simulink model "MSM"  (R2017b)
settings: Solver=FixedStepDiscrete  StartTime=0.0  StopTime=10.0  FixedStep=0.01  RelTol=1e-3  EnableMultiTasking=on
undefined symbols (not defined in the file): ASWTYPE_FALSE, ASWTYPE_TRUE, CcMSM_NetWorkRlsTi_ms, CcMSM_PreShutTi_ms, CcMSM_RadySleepFltTi_ms, CcMSM_SelfCheckFltThrhd_numb, CcMSM_ShutdownToSleepTi_ms, CcMSM_ShutdownToStbTi_ms, CcMSM_StandbyRunTime_ms, CcMSM_StbToPreShutDlyTi_ms, Enum_CTCCtrCtlState, Enum_ISPBsicSysMod, Enum_ISPNetWkUpSt, Enum_MSMBMUState, Enum_VDPDriveRqst, MSM_RUNTIME_MS, WAKEUP_DEFAULT
libraries: AIWAYS_Powertrain_BMS_lib x18

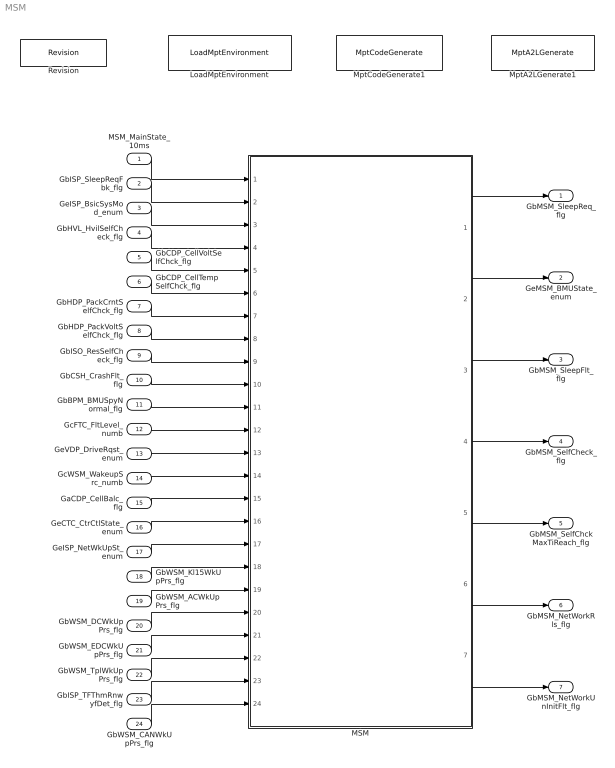
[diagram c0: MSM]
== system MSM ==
  MSM_MainState_10ms : Inport
  GbISP_SleepReqFbk_flg : Inport  Port=2
  GeISP_BsicSysMod_enum : Inport  Port=3
  GbHVL_HvilSelfCheck_flg : Inport  Port=4
  GbCDP_CellVoltSelfChck_flg : Inport  Port=5
  GbCDP_CellTempSelfChck_flg : Inport  Port=6
  GbHDP_PackCrntSelfChck_flg : Inport  Port=7
  GbHDP_PackVoltSelfChck_flg : Inport  Port=8
  GbISO_ResSelfCheck_flg : Inport  Port=9
  GbCSH_CrashFlt_flg : Inport  Port=10
  GbBPM_BMUSpyNormal_flg : Inport  Port=11
  GcFTC_FltLevel_numb : Inport  Port=12
  GeVDP_DriveRqst_enum : Inport  Port=13
  GcWSM_WakeupSrc_numb : Inport  Port=14
  GaCDP_CellBalc_flg : Inport  Port=15
  GeCTC_CtrCtlState_enum : Inport  Port=16
  GeISP_NetWkUpSt_enum : Inport  Port=17
  GbWSM_Kl15WkUpPrs_flg : Inport  Port=18
  GbWSM_ACWkUpPrs_flg : Inport  Port=19
  GbWSM_DCWkUpPrs_flg : Inport  Port=20
  GbWSM_EDCWkUpPrs_flg : Inport  Port=21
  GbWSM_TplWkUpPrs_flg : Inport  Port=22
  GbISP_TFThmRnwyfDet_flg : Inport  Port=23
  GbWSM_CANWkUpPrs_flg : Inport  Port=24
  LoadMptEnvironment : AIWAYS_Powertrain_BMS_lib/Config/LoadMptEnvironment  ProjectName=Comm  SuppierID=NewPlatformUAES
  MSM : Subsystem
  MptA2LGenerate1 : AIWAYS_Powertrain_BMS_lib/Config/MptA2LGenerate  SystemSampleTime=-1
  MptCodeGenerate1 : AIWAYS_Powertrain_BMS_lib/Config/MptCodeGenerate  SystemSampleTime=-1
  Revision : AIWAYS_Powertrain_BMS_lib/Config/Revision  curVersion='M108C103'  newVersion='M108C103'
  GbMSM_SleepReq_flg : Outport
  GeMSM_BMUState_enum : Outport  Port=2
  GbMSM_SleepFlt_flg : Outport  Port=3
  GbMSM_SelfCheck_flg : Outport  Port=4
  GbMSM_SelfChckMaxTiReach_flg : Outport  Port=5
  GbMSM_NetWorkRls_flg : Outport  Port=6
  GbMSM_NetWorkUnInitFlt_flg : Outport  Port=7
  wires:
  MSM_MainState_10ms/1 -> MSM/1(MSM_MainState_10ms)
  GbISP_SleepReqFbk_flg/1 -> MSM/2(GbISP_SleepReqFbk_flg)
  GeISP_BsicSysMod_enum/1 -> MSM/3(GeISP_BsicSysMod_enum)
  GbHVL_HvilSelfCheck_flg/1 -> MSM/4(GbHVL_HvilSelfCheck_flg)
  GbCDP_CellVoltSelfChck_flg/1 -> MSM/5(GbCDP_CellVoltSelfChck_flg)
  GbCDP_CellTempSelfChck_flg/1 -> MSM/6(GbCDP_CellTempSelfChck_flg)
  GbHDP_PackCrntSelfChck_flg/1 -> MSM/7(GbHDP_PackCrntSelfChck_flg)
  GbHDP_PackVoltSelfChck_flg/1 -> MSM/8(GbHDP_PackVoltSelfChck_flg)
  GbISO_ResSelfCheck_flg/1 -> MSM/9(GbISO_ResSelfCheck_flg)
  GbCSH_CrashFlt_flg/1 -> MSM/10(GbCSH_CrashFlt_flg)
  GbBPM_BMUSpyNormal_flg/1 -> MSM/11(GbBPM_BMUSpyNormal_flg)
  GcFTC_FltLevel_numb/1 -> MSM/12(GcFTC_FltLevel_numb)
  GeVDP_DriveRqst_enum/1 -> MSM/13(GeVDP_DriveRqst_enum)
  GcWSM_WakeupSrc_numb/1 -> MSM/14(GcWSM_WakeupSrc_numb)
  GaCDP_CellBalc_flg/1 -> MSM/15(GaCDP_CellBalc_flg)
  GeCTC_CtrCtlState_enum/1 -> MSM/16(GeCTC_CtrCtlState_enum)
  GbWSM_Kl15WkUpPrs_flg/1 -> MSM/18(GbWSM_Kl15WkUpPrs_flg)
  GbWSM_ACWkUpPrs_flg/1 -> MSM/19(GbWSM_ACWkUpPrs_flg)
  GbWSM_DCWkUpPrs_flg/1 -> MSM/20(GbWSM_DCWkUpPrs_flg)
  GbWSM_EDCWkUpPrs_flg/1 -> MSM/21(GbWSM_EDCWkUpPrs_flg)
  MSM/1(GbMSM_SleepReq_flg) -> GbMSM_SleepReq_flg/1
  MSM/2(GeMSM_BMUState_enum) -> GeMSM_BMUState_enum/1
  MSM/3(GbMSM_SleepFlt_flg) -> GbMSM_SleepFlt_flg/1
  MSM/4(GbMSM_SelfCheck_flg) -> GbMSM_SelfCheck_flg/1
  MSM/5(GbMSM_SelfChckMaxTiReach_flg) -> GbMSM_SelfChckMaxTiReach_flg/1
  MSM/6(GbMSM_NetWorkRls_flg) -> GbMSM_NetWorkRls_flg/1
  MSM/7(GbMSM_NetWorkUnInitFlt_flg) -> GbMSM_NetWorkUnInitFlt_flg/1
  GbWSM_TplWkUpPrs_flg/1 -> MSM/22(GbWSM_TplWkUpPrs_flg)
  GbISP_TFThmRnwyfDet_flg/1 -> MSM/23(GbISP_TFThmRnwyfDet_flg)
  GbWSM_CANWkUpPrs_flg/1 -> MSM/24(GbWSM_CANWkUpPrs_flg)
  GeISP_NetWkUpSt_enum/1 -> MSM/17(GeISP_NetWkUpSt_enum)

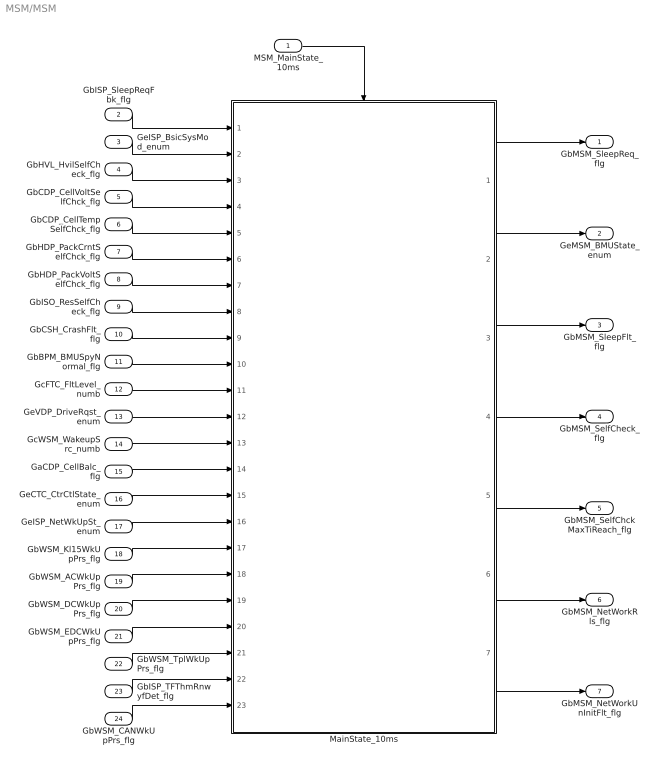
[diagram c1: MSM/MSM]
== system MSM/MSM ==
  MSM_MainState_10ms : Inport
  GbISP_SleepReqFbk_flg : Inport  Port=2
  GeISP_BsicSysMod_enum : Inport  Port=3
  GbHVL_HvilSelfCheck_flg : Inport  Port=4
  GbCDP_CellVoltSelfChck_flg : Inport  Port=5
  GbCDP_CellTempSelfChck_flg : Inport  Port=6
  GbHDP_PackCrntSelfChck_flg : Inport  Port=7
  GbHDP_PackVoltSelfChck_flg : Inport  Port=8
  GbISO_ResSelfCheck_flg : Inport  Port=9
  GbCSH_CrashFlt_flg : Inport  Port=10
  GbBPM_BMUSpyNormal_flg : Inport  Port=11
  GcFTC_FltLevel_numb : Inport  Port=12
  GeVDP_DriveRqst_enum : Inport  Port=13
  GcWSM_WakeupSrc_numb : Inport  Port=14
  GaCDP_CellBalc_flg : Inport  Port=15
  GeCTC_CtrCtlState_enum : Inport  Port=16
  GeISP_NetWkUpSt_enum : Inport  Port=17
  GbWSM_Kl15WkUpPrs_flg : Inport  Port=18
  GbWSM_ACWkUpPrs_flg : Inport  Port=19
  GbWSM_DCWkUpPrs_flg : Inport  Port=20
  GbWSM_EDCWkUpPrs_flg : Inport  Port=21
  GbWSM_TplWkUpPrs_flg : Inport  Port=22
  GbISP_TFThmRnwyfDet_flg : Inport  Port=23
  GbWSM_CANWkUpPrs_flg : Inport  Port=24
  MainState_10ms : Subsystem
  GbMSM_SleepReq_flg : Outport
  GeMSM_BMUState_enum : Outport  Port=2
  GbMSM_SleepFlt_flg : Outport  Port=3
  GbMSM_SelfCheck_flg : Outport  Port=4
  GbMSM_SelfChckMaxTiReach_flg : Outport  Port=5
  GbMSM_NetWorkRls_flg : Outport  Port=6
  GbMSM_NetWorkUnInitFlt_flg : Outport  Port=7
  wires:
  MSM_MainState_10ms/1 -> MainState_10ms/Trigger
  GbISP_SleepReqFbk_flg/1 -> MainState_10ms/1(GbISP_SleepReqFbk_flg)
  GeISP_BsicSysMod_enum/1 -> MainState_10ms/2(GeISP_BsicSysMod_enum)
  GbHVL_HvilSelfCheck_flg/1 -> MainState_10ms/3(GbHVL_HvilSelfCheck_flg)
  GbCDP_CellVoltSelfChck_flg/1 -> MainState_10ms/4(GbCDP_CellVoltSelfChck_flg)
  GbCDP_CellTempSelfChck_flg/1 -> MainState_10ms/5(GbCDP_CellTempSelfChck_flg)
  GbHDP_PackCrntSelfChck_flg/1 -> MainState_10ms/6(GbHDP_PackCrntSelfChck_flg)
  GbHDP_PackVoltSelfChck_flg/1 -> MainState_10ms/7(GbHDP_PackVoltSelfChck_flg)
  GbISO_ResSelfCheck_flg/1 -> MainState_10ms/8(GbISO_ResSelfCheck_flg)
  GbCSH_CrashFlt_flg/1 -> MainState_10ms/9(GbCSH_CrashFlt_flg)
  GbBPM_BMUSpyNormal_flg/1 -> MainState_10ms/10(GbBPM_BMUSpyNormal_flg)
  GcFTC_FltLevel_numb/1 -> MainState_10ms/11(GcFTC_FltLevel_numb)
  GeVDP_DriveRqst_enum/1 -> MainState_10ms/12(GeVDP_DriveRqst_enum)
  GcWSM_WakeupSrc_numb/1 -> MainState_10ms/13(GcWSM_WakeupSrc_numb)
  GaCDP_CellBalc_flg/1 -> MainState_10ms/14(GaCDP_CellBalc_flg)
  GeCTC_CtrCtlState_enum/1 -> MainState_10ms/15(GeCTC_CtrCtlState_enum)
  GbWSM_Kl15WkUpPrs_flg/1 -> MainState_10ms/17(GbWSM_Kl15WkUpPrs_flg)
  GbWSM_ACWkUpPrs_flg/1 -> MainState_10ms/18(GbWSM_ACWkUpPrs_flg)
  GbWSM_DCWkUpPrs_flg/1 -> MainState_10ms/19(GbWSM_DCWkUpPrs_flg)
  GbWSM_EDCWkUpPrs_flg/1 -> MainState_10ms/20(GbWSM_EDCWkUpPrs_flg)
  MainState_10ms/4(GbMSM_SelfCheck_flg) -> GbMSM_SelfCheck_flg/1
  MainState_10ms/7(GbMSM_NetWorkUnInitFlt_flg) -> GbMSM_NetWorkUnInitFlt_flg/1
  MainState_10ms/6(GbMSM_NetWorkRls_flg) -> GbMSM_NetWorkRls_flg/1
  MainState_10ms/2(GeMSM_BMUState_enum) -> GeMSM_BMUState_enum/1
  MainState_10ms/3(GbMSM_SleepFlt_flg) -> GbMSM_SleepFlt_flg/1
  MainState_10ms/1(GbMSM_SleepReq_flg) -> GbMSM_SleepReq_flg/1
  MainState_10ms/5(GbMSM_SelfChckMaxTiReach_flg) -> GbMSM_SelfChckMaxTiReach_flg/1
  GbWSM_TplWkUpPrs_flg/1 -> MainState_10ms/21(GbWSM_TplWkUpPrs_flg)
  GbISP_TFThmRnwyfDet_flg/1 -> MainState_10ms/22(GbISP_TFThmRnwyfDet_flg)
  GbWSM_CANWkUpPrs_flg/1 -> MainState_10ms/23(GbWSM_CANWkUpPrs_flg)
  GeISP_NetWkUpSt_enum/1 -> MainState_10ms/16(GeISP_NetWkUpSt_enum)

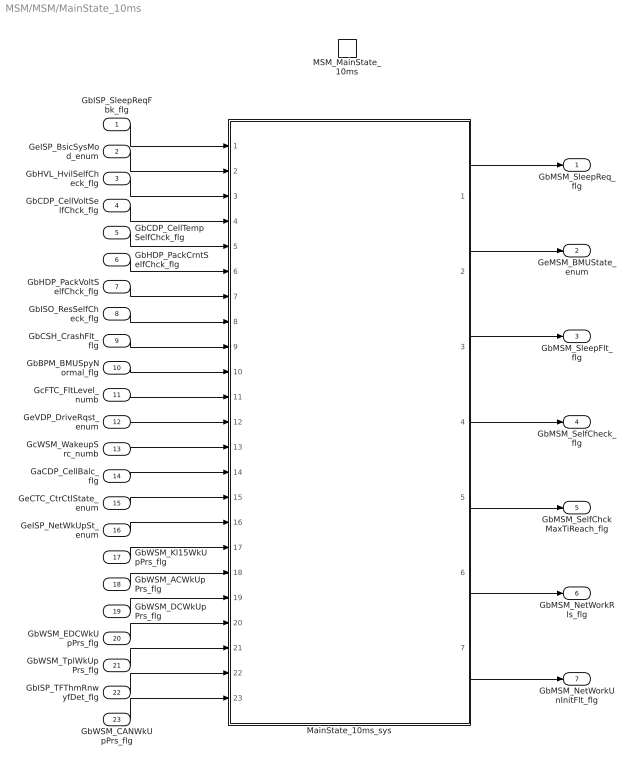
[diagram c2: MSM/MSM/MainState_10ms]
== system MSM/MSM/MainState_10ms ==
  GbISP_SleepReqFbk_flg : Inport
  GeISP_BsicSysMod_enum : Inport  Port=2
  GbHVL_HvilSelfCheck_flg : Inport  Port=3
  GbCDP_CellVoltSelfChck_flg : Inport  Port=4
  GbCDP_CellTempSelfChck_flg : Inport  Port=5
  GbHDP_PackCrntSelfChck_flg : Inport  Port=6
  GbHDP_PackVoltSelfChck_flg : Inport  Port=7
  GbISO_ResSelfCheck_flg : Inport  Port=8
  GbCSH_CrashFlt_flg : Inport  Port=9
  GbBPM_BMUSpyNormal_flg : Inport  Port=10
  GcFTC_FltLevel_numb : Inport  Port=11
  GeVDP_DriveRqst_enum : Inport  Port=12
  GcWSM_WakeupSrc_numb : Inport  Port=13
  GaCDP_CellBalc_flg : Inport  Port=14
  GeCTC_CtrCtlState_enum : Inport  Port=15
  GeISP_NetWkUpSt_enum : Inport  Port=16
  GbWSM_Kl15WkUpPrs_flg : Inport  Port=17
  GbWSM_ACWkUpPrs_flg : Inport  Port=18
  GbWSM_DCWkUpPrs_flg : Inport  Port=19
  GbWSM_EDCWkUpPrs_flg : Inport  Port=20
  GbWSM_TplWkUpPrs_flg : Inport  Port=21
  GbISP_TFThmRnwyfDet_flg : Inport  Port=22
  GbWSM_CANWkUpPrs_flg : Inport  Port=23
  MSM_MainState_10ms : TriggerPort  TriggerType=function-call  VariantControl=(inherit)
  MainState_10ms_sys : Subsystem
  GbMSM_SleepReq_flg : Outport
  GeMSM_BMUState_enum : Outport  Port=2
  GbMSM_SleepFlt_flg : Outport  Port=3
  GbMSM_SelfCheck_flg : Outport  Port=4
  GbMSM_SelfChckMaxTiReach_flg : Outport  Port=5
  GbMSM_NetWorkRls_flg : Outport  Port=6
  GbMSM_NetWorkUnInitFlt_flg : Outport  Port=7
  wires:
  GbISP_SleepReqFbk_flg/1 -> MainState_10ms_sys/1(GbISP_SleepReqFbk_flg)
  GeISP_BsicSysMod_enum/1 -> MainState_10ms_sys/2(GeISP_BsicSysMod_enum)
  GbHVL_HvilSelfCheck_flg/1 -> MainState_10ms_sys/3(GbHVL_HvilSelfCheck_flg)
  GbCDP_CellVoltSelfChck_flg/1 -> MainState_10ms_sys/4(GbCDP_CellVoltSelfChck_flg)
  GbCDP_CellTempSelfChck_flg/1 -> MainState_10ms_sys/5(GbCDP_CellTempSelfChck_flg)
  GbHDP_PackCrntSelfChck_flg/1 -> MainState_10ms_sys/6(GbHDP_PackCrntSelfChck_flg)
  GbHDP_PackVoltSelfChck_flg/1 -> MainState_10ms_sys/7(GbHDP_PackVoltSelfChck_flg)
  GbISO_ResSelfCheck_flg/1 -> MainState_10ms_sys/8(GbISO_ResSelfCheck_flg)
  GbCSH_CrashFlt_flg/1 -> MainState_10ms_sys/9(GbCSH_CrashFlt_flg)
  GbBPM_BMUSpyNormal_flg/1 -> MainState_10ms_sys/10(GbBPM_BMUSpyNormal_flg)
  GcFTC_FltLevel_numb/1 -> MainState_10ms_sys/11(GcFTC_FltLevel_numb)
  GeVDP_DriveRqst_enum/1 -> MainState_10ms_sys/12(GeVDP_DriveRqst_enum)
  GcWSM_WakeupSrc_numb/1 -> MainState_10ms_sys/13(GcWSM_WakeupSrc_numb)
  GaCDP_CellBalc_flg/1 -> MainState_10ms_sys/14(GaCDP_CellBalc_flg)
  GeCTC_CtrCtlState_enum/1 -> MainState_10ms_sys/15(GeCTC_CtrCtlState_enum)
  GbWSM_Kl15WkUpPrs_flg/1 -> MainState_10ms_sys/17(GbWSM_Kl15WkUpPrs_flg)
  GbWSM_ACWkUpPrs_flg/1 -> MainState_10ms_sys/18(GbWSM_ACWkUpPrs_flg)
  GbWSM_DCWkUpPrs_flg/1 -> MainState_10ms_sys/19(GbWSM_DCWkUpPrs_flg)
  GbWSM_EDCWkUpPrs_flg/1 -> MainState_10ms_sys/20(GbWSM_EDCWkUpPrs_flg)
  MainState_10ms_sys/1(GbMSM_SleepReq_flg) -> GbMSM_SleepReq_flg/1
  MainState_10ms_sys/2(GeMSM_BMUState_enum) -> GeMSM_BMUState_enum/1
  MainState_10ms_sys/3(GbMSM_SleepFlt_flg) -> GbMSM_SleepFlt_flg/1
  MainState_10ms_sys/4(GbMSM_SelfCheck_flg) -> GbMSM_SelfCheck_flg/1
  MainState_10ms_sys/5(GbMSM_SelfChckMaxTiReach_flg) -> GbMSM_SelfChckMaxTiReach_flg/1
  MainState_10ms_sys/6(GbMSM_NetWorkRls_flg) -> GbMSM_NetWorkRls_flg/1
  MainState_10ms_sys/7(GbMSM_NetWorkUnInitFlt_flg) -> GbMSM_NetWorkUnInitFlt_flg/1
  GbWSM_TplWkUpPrs_flg/1 -> MainState_10ms_sys/21(GbWSM_TplWkUpPrs_flg)
  GbISP_TFThmRnwyfDet_flg/1 -> MainState_10ms_sys/22(GbISP_TFThmRnwyfDet_flg)
  GbWSM_CANWkUpPrs_flg/1 -> MainState_10ms_sys/23(GbWSM_CANWkUpPrs_flg)
  GeISP_NetWkUpSt_enum/1 -> MainState_10ms_sys/16(GeISP_NetWkUpSt_enum)

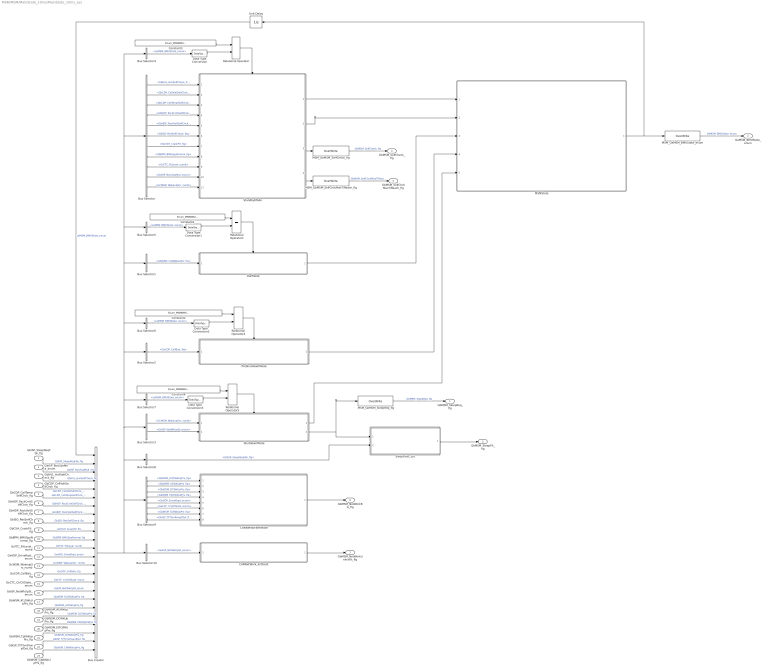
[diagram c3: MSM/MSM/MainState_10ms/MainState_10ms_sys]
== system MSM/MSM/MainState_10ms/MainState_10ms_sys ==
  GbISP_SleepReqFbk_flg : Inport
  GeISP_BsicSysMod_enum : Inport  Port=2
  GbHVL_HvilSelfCheck_flg : Inport  Port=3
  GbCDP_CellVoltSelfChck_flg : Inport  Port=4
  GbCDP_CellTempSelfChck_flg : Inport  Port=5
  GbHDP_PackCrntSelfChck_flg : Inport  Port=6
  GbHDP_PackVoltSelfChck_flg : Inport  Port=7
  GbISO_ResSelfCheck_flg : Inport  Port=8
  GbCSH_CrashFlt_flg : Inport  Port=9
  GbBPM_BMUSpyNormal_flg : Inport  Port=10
  GcFTC_FltLevel_numb : Inport  Port=11
  GeVDP_DriveRqst_enum : Inport  Port=12
  GcWSM_WakeupSrc_numb : Inport  Port=13
  GaCDP_CellBalc_flg : Inport  Port=14
  GeCTC_CtrCtlState_enum : Inport  Port=15
  GeISP_NetWkUpSt_enum : Inport  Port=16
  GbWSM_Kl15WkUpPrs_flg : Inport  Port=17
  GbWSM_ACWkUpPrs_flg : Inport  Port=18
  GbWSM_DCWkUpPrs_flg : Inport  Port=19
  GbWSM_EDCWkUpPrs_flg : Inport  Port=20
  GbWSM_TplWkUpPrs_flg : Inport  Port=21
  GbISP_TFThmRnwyfDet_flg : Inport  Port=22
  GbWSM_CANWkUpPrs_flg : Inport  Port=23
  Bus Creator : BusCreator  Inputs=24
  Bus Selector : BusSelector  OutputSignals=GbHVL_HvilSelfCheck_flg,GbCDP_CellVoltSelfChck_flg,GbCDP_CellTempSelfChck_flg,GbHDP_PackCrntSelfChck_flg,GbHDP_PackVoltSelfChck_flg,GbISO_ResSelfCheck_flg,GbCSH_CrashFlt_flg,GbBPM_BMUSpyNormal_flg,GcFTC_FltLevel_numb,GeISP_BsicSysMod_enum,GcWSM_WakeupSrc_numb
  Bus Selector1 : BusSelector  OutputSignals=GbWSM_CANWkUpPrs_flg
  Bus Selector10 : BusSelector  OutputSignals=GeISP_NetWkUpSt_enum
  Bus Selector2 : BusSelector  OutputSignals=GaCDP_CellBalc_flg
  Bus Selector3 : BusSelector  OutputSignals=GcWSM_WakeupSrc_numb,GeISP_NetWkUpSt_enum
  Bus Selector{4..7} (4 alike) : BusSelector  OutputSignals=LeMSM_BMUState_enum
  Bus Selector8 : BusSelector  OutputSignals=GbISP_SleepReqFbk_flg
  Bus Selector9 : BusSelector  OutputSignals=GbWSM_Kl15WkUpPrs_flg,GbWSM_ACWkUpPrs_flg,GbWSM_DCWkUpPrs_flg,GbWSM_EDCWkUpPrs_flg,GeVDP_DriveRqst_enum,GeCTC_CtrCtlState_enum,GbWSM_TplWkUpPrs_flg,GbISP_TFThmRnwyfDet_flg
  CANNetWorkRelease : Subsystem
  CANNetWork_InitFault : Subsystem
  Constant1 : Constant  Value=Enum_MSMBMUState.Enum_MSMBMUState_Run
  Constant2 : Constant  Value=Enum_MSMBMUState.Enum_MSMBMUState_PreShutdown
  Constant3 : Constant  Value=Enum_MSMBMUState.Enum_MSMBMUState_Standby
  Constant4 : Constant  Value=Enum_MSMBMUState.Enum_MSMBMUState_Shutdown
  Data Type Conversion{,1..3} (4 alike) : DataTypeConversion
  MSMState : Stateflow chart  TreatAsAtomicUnit=on
  MSM_GbMSM_SelfChckMaxTiReach_flg : AIWAYS_Powertrain_BMS_lib/Signals/OverWrite  OverWrite_Value=CbMSM_SelfChckMaxTiReachOvr_flg  OverWrite_flag=CbMSM_SelfChckMaxTiReachOvrSwt_flg
  MSM_GbMSM_SelfCheck_flg : AIWAYS_Powertrain_BMS_lib/Signals/OverWrite  OverWrite_Value=CbMSM_SelfCheckOvr_flg  OverWrite_flag=CbMSM_SelfCheckOvrSwt_flg
  MSM_GbMSM_SleepReq_flg : AIWAYS_Powertrain_BMS_lib/Signals/OverWrite  OverWrite_Value=CbMSM_SleepReqOvr_flg  OverWrite_flag=CbMSM_SleepReqOvrSwt_flg
  MSM_GeMSM_BMUState_enum : AIWAYS_Powertrain_BMS_lib/Signals/OverWrite  OverWrite_Value=CeMSM_BMUStateOvr_enum  OverWrite_flag=CbMSM_BMUStateOvrSwt_flg
  PreShutdownMode : Subsystem  TreatAsAtomicUnit=on
  Relational Operator{,1,4..5} (4 alike) : RelationalOperator  Operator===  OutDataTypeStr=boolean
  RunMode : Subsystem  TreatAsAtomicUnit=on
  ShutdownMode : Subsystem  TreatAsAtomicUnit=on
  SleepFault_sys : Subsystem
  StandbyMode : Subsystem  TreatAsAtomicUnit=on
  Unit Delay : UnitDelay  SampleTime=-1
  GbMSM_SleepReq_flg : Outport
  GeMSM_BMUState_enum : Outport  Port=2
  GbMSM_SleepFlt_flg : Outport  Port=3
  GbMSM_SelfCheck_flg : Outport  Port=4
  GbMSM_SelfChckMaxTiReach_flg : Outport  Port=5
  GbMSM_NetWorkRls_flg : Outport  Port=6
  GbMSM_NetWorkUnInitFlt_flg : Outport  Port=7
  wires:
  GbISP_SleepReqFbk_flg/1 -> Bus Creator/2  "GbISP_SleepReqFbk_flg"
  GeISP_BsicSysMod_enum/1 -> Bus Creator/3  "GeISP_BsicSysMod_enum"
  GbHVL_HvilSelfCheck_flg/1 -> Bus Creator/4  "GbHVL_HvilSelfCheck_flg"
  GbCDP_CellVoltSelfChck_flg/1 -> Bus Creator/5  "GbCDP_CellVoltSelfChck_flg"
  GbCDP_CellTempSelfChck_flg/1 -> Bus Creator/6  "GbCDP_CellTempSelfChck_flg"
  GbHDP_PackCrntSelfChck_flg/1 -> Bus Creator/7  "GbHDP_PackCrntSelfChck_flg"
  GbHDP_PackVoltSelfChck_flg/1 -> Bus Creator/8  "GbHDP_PackVoltSelfChck_flg"
  GbISO_ResSelfCheck_flg/1 -> Bus Creator/9  "GbISO_ResSelfCheck_flg"
  GbCSH_CrashFlt_flg/1 -> Bus Creator/10  "GbCSH_CrashFlt_flg"
  GbBPM_BMUSpyNormal_flg/1 -> Bus Creator/11  "GbBPM_BMUSpyNormal_flg"
  GcFTC_FltLevel_numb/1 -> Bus Creator/12  "GcFTC_FltLevel_numb"
  GeVDP_DriveRqst_enum/1 -> Bus Creator/13  "GeVDP_DriveRqst_enum"
  GcWSM_WakeupSrc_numb/1 -> Bus Creator/14  "GcWSM_WakeupSrc_numb"
  GaCDP_CellBalc_flg/1 -> Bus Creator/15  "GaCDP_CellBalc_flg"
  GeCTC_CtrCtlState_enum/1 -> Bus Creator/16  "GeCTC_CtrCtlState_enum"
  Bus Creator/1 -> Bus Selector8/1, Bus Selector4/1, Bus Selector/1, Bus Selector5/1, Bus Selector1/1, Bus Selector6/1, Bus Selector2/1, Bus Selector7/1, Bus Selector3/1, Bus Selector9/1, Bus Selector10/1
  Bus Selector2/1 -> PreShutdownMode/1(GaCDP_CellBalc_flg)  "<GaCDP_CellBalc_flg>"
  Bus Selector3/1 -> ShutdownMode/1(GcWSM_WakeupSrc_numb)  "<GcWSM_WakeupSrc_numb>"
  StandbyMode/1(LbMSM_StandbyToRun_flg) -> MSMState/1(LbMSM_StandbyToRun_flg)
  StandbyMode/2(LbMSM_StbToPreShut_flg) -> MSMState/2(LbMSM_StbToPreShut_flg)
  RunMode/1(LbMSM_RunToPreShut_flg) -> MSMState/3(LbMSM_RunToPreShut_flg)
  PreShutdownMode/1(LbMSM_PreShutToShut_flg) -> MSMState/4(LbMSM_PreShutToShut_flg)
  ShutdownMode/1(LbMSM_ShutdownToStb_flg) -> MSMState/5(LbMSM_ShutdownToStb_flg)
  MSMState/1(GeMSM_BMUState_enum) -> Unit Delay/1, MSM_GeMSM_BMUState_enum/1
  Relational Operator/1 -> StandbyMode/Enable
  Unit Delay/1 -> Bus Creator/1  "LeMSM_BMUState_enum"
  Constant3/1 -> Relational Operator/1
  Bus Selector4/1 -> Data Type Conversion/1  "<LeMSM_BMUState_enum>"
  Data Type Conversion/1 -> Relational Operator/2
  Bus Selector5/1 -> Data Type Conversion1/1  "<LeMSM_BMUState_enum>"
  Constant1/1 -> Relational Operator1/1
  Relational Operator1/1 -> RunMode/Enable
  Data Type Conversion1/1 -> Relational Operator1/2
  Relational Operator4/1 -> PreShutdownMode/Enable
  Bus Selector6/1 -> Data Type Conversion2/1  "<LeMSM_BMUState_enum>"
  Constant2/1 -> Relational Operator4/1
  Data Type Conversion2/1 -> Relational Operator4/2
  Relational Operator5/1 -> ShutdownMode/Enable
  Bus Selector7/1 -> Data Type Conversion3/1  "<LeMSM_BMUState_enum>"
  Constant4/1 -> Relational Operator5/1
  Data Type Conversion3/1 -> Relational Operator5/2
  MSM_GeMSM_BMUState_enum/1 -> GeMSM_BMUState_enum/1  "GeMSM_BMUState_enum"
  Bus Selector/1 -> StandbyMode/1(GbHVL_HvilSelfCheck_flg)  "<GbHVL_HvilSelfCheck_flg>"
  Bus Selector/2 -> StandbyMode/2(GbCDP_CellVoltSelfChck_flg)  "<GbCDP_CellVoltSelfChck_flg>"
  Bus Selector/3 -> StandbyMode/3(GbCDP_CellTempSelfChck_flg)  "<GbCDP_CellTempSelfChck_flg>"
  Bus Selector/4 -> StandbyMode/4(GbHDP_PackCrntSelfChck_flg)  "<GbHDP_PackCrntSelfChck_flg>"
  Bus Selector/5 -> StandbyMode/5(GbHDP_PackVoltSelfChck_flg)  "<GbHDP_PackVoltSelfChck_flg>"
  Bus Selector/6 -> StandbyMode/6(GbISO_ResSelfCheck_flg)  "<GbISO_ResSelfCheck_flg>"
  Bus Selector/7 -> StandbyMode/7(GbCSH_CrashFlt_flg)  "<GbCSH_CrashFlt_flg>"
  Bus Selector/8 -> StandbyMode/8(GbBPM_BMUSpyNormal_flg)  "<GbBPM_BMUSpyNormal_flg>"
  Bus Selector/9 -> StandbyMode/9(GcFTC_FltLevel_numb)  "<GcFTC_FltLevel_numb>"
  Bus Selector/10 -> StandbyMode/10(GeISP_BsicSysMod_enum)  "<GeISP_BsicSysMod_enum>"
  Bus Selector/11 -> StandbyMode/11(GcWSM_WakeupSrc_numb)  "<GcWSM_WakeupSrc_numb>"
  Bus Selector3/2 -> ShutdownMode/2(GeISP_NetWkUpSt_enum)  "<GeISP_NetWkUpSt_enum>"
  MSM_GbMSM_SleepReq_flg/1 -> GbMSM_SleepReq_flg/1  "GbMSM_SleepReq_flg"
  ShutdownMode/2(LbMSM_SleepReq_flg) -> SleepFault_sys/1(LbMSM_SleepReq_flg), MSM_GbMSM_SleepReq_flg/1
  SleepFault_sys/1(GbMSM_SleepFlt_flg) -> GbMSM_SleepFlt_flg/1
  Bus Selector8/1 -> SleepFault_sys/2(GbISP_SleepReqFbk_flg)  "<GbISP_SleepReqFbk_flg>"
  MSM_GbMSM_SelfCheck_flg/1 -> GbMSM_SelfCheck_flg/1  "GbMSM_SelfCheck_flg"
  StandbyMode/3(LbMSM_SelfCheck_flg) -> MSM_GbMSM_SelfCheck_flg/1
  MSM_GbMSM_SelfChckMaxTiReach_flg/1 -> GbMSM_SelfChckMaxTiReach_flg/1  "GbMSM_SelfChckMaxTiReach_flg"
  StandbyMode/4(LbMSM_SelfChckMaxTiReach_flg) -> MSM_GbMSM_SelfChckMaxTiReach_flg/1
  Bus Selector1/1 -> RunMode/1(GbWSM_CANWkUpPrs_flg)  "<GbWSM_CANWkUpPrs_flg>"
  GbWSM_Kl15WkUpPrs_flg/1 -> Bus Creator/18  "GbWSM_Kl15WkUpPrs_flg"
  GbWSM_ACWkUpPrs_flg/1 -> Bus Creator/19  "GbWSM_ACWkUpPrs_flg"
  GbWSM_DCWkUpPrs_flg/1 -> Bus Creator/20  "GbWSM_DCWkUpPrs_flg"
  GbWSM_EDCWkUpPrs_flg/1 -> Bus Creator/21  "GbWSM_EDCWkUpPrs_flg"
  CANNetWorkRelease/1(GbMSM_NetWorkRls_flg) -> GbMSM_NetWorkRls_flg/1
  Bus Selector10/1 -> CANNetWork_InitFault/1(GeISP_NetWkUpSt_enum)  "<GeISP_NetWkUpSt_enum>"
  CANNetWork_InitFault/1(GbMSM_NetWorkUnInitFlt_flg) -> GbMSM_NetWorkUnInitFlt_flg/1
  Bus Selector9/1 -> CANNetWorkRelease/1(GbWSM_Kl15WkUpPrs_flg)  "<GbWSM_Kl15WkUpPrs_flg>"
  Bus Selector9/2 -> CANNetWorkRelease/2(GbWSM_ACWkUpPrs_flg)  "<GbWSM_ACWkUpPrs_flg>"
  Bus Selector9/3 -> CANNetWorkRelease/3(GbWSM_DCWkUpPrs_flg)  "<GbWSM_DCWkUpPrs_flg>"
  Bus Selector9/4 -> CANNetWorkRelease/4(GbWSM_EDCWkUpPrs_flg)  "<GbWSM_EDCWkUpPrs_flg>"
  Bus Selector9/5 -> CANNetWorkRelease/5(GeVDP_DriveRqst_enum)  "<GeVDP_DriveRqst_enum>"
  Bus Selector9/6 -> CANNetWorkRelease/6(GeCTC_CtrCtlState_enum)  "<GeCTC_CtrCtlState_enum>"
  GbWSM_TplWkUpPrs_flg/1 -> Bus Creator/22  "GbWSM_TplWkUpPrs_flg"
  GbISP_TFThmRnwyfDet_flg/1 -> Bus Creator/23  "GbISP_TFThmRnwyfDet_flg"
  Bus Selector9/7 -> CANNetWorkRelease/7(GbWSM_TplWkUpPrs_flg)  "<GbWSM_TplWkUpPrs_flg>"
  Bus Selector9/8 -> CANNetWorkRelease/8(GbISP_TFThmRnwyfDet_flg)  "<GbISP_TFThmRnwyfDet_flg>"
  GbWSM_CANWkUpPrs_flg/1 -> Bus Creator/24  "GbWSM_CANWkUpPrs_flg"
  GeISP_NetWkUpSt_enum/1 -> Bus Creator/17  "GeISP_NetWkUpSt_enum"

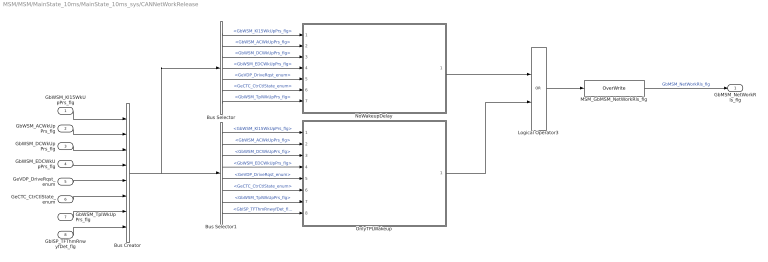
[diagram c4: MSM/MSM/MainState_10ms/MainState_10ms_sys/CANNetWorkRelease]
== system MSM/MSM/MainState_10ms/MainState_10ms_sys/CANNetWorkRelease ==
  GbWSM_Kl15WkUpPrs_flg : Inport
  GbWSM_ACWkUpPrs_flg : Inport  Port=2
  GbWSM_DCWkUpPrs_flg : Inport  Port=3
  GbWSM_EDCWkUpPrs_flg : Inport  Port=4
  GeVDP_DriveRqst_enum : Inport  Port=5
  GeCTC_CtrCtlState_enum : Inport  Port=6
  GbWSM_TplWkUpPrs_flg : Inport  Port=7
  GbISP_TFThmRnwyfDet_flg : Inport  Port=8
  Bus Creator : BusCreator  Inputs=8
  Bus Selector : BusSelector  OutputSignals=GbWSM_Kl15WkUpPrs_flg,GbWSM_ACWkUpPrs_flg,GbWSM_DCWkUpPrs_flg,GbWSM_EDCWkUpPrs_flg,GeVDP_DriveRqst_enum,GeCTC_CtrCtlState_enum,GbWSM_TplWkUpPrs_flg
  Bus Selector1 : BusSelector  OutputSignals=GbWSM_Kl15WkUpPrs_flg,GbWSM_ACWkUpPrs_flg,GbWSM_DCWkUpPrs_flg,GbWSM_EDCWkUpPrs_flg,GeVDP_DriveRqst_enum,GeCTC_CtrCtlState_enum,GbWSM_TplWkUpPrs_flg,GbISP_TFThmRnwyfDet_flg
  Logical Operator3 : Logic  Operator=OR  AllPortsSameDT=off  OutDataTypeStr=boolean
  MSM_GbMSM_NetWorkRls_flg : AIWAYS_Powertrain_BMS_lib/Signals/OverWrite  OverWrite_Value=CbMSM_NetWorkRlsOvr_flg  OverWrite_flag=CbMSM_NetWorkRlsOvrSwt_flg
  NoWakeupDelay : Subsystem
  OnlyTPLWakeup : Subsystem
  GbMSM_NetWorkRls_flg : Outport
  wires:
  Logical Operator3/1 -> MSM_GbMSM_NetWorkRls_flg/1
  MSM_GbMSM_NetWorkRls_flg/1 -> GbMSM_NetWorkRls_flg/1  "GbMSM_NetWorkRls_flg"
  GbWSM_Kl15WkUpPrs_flg/1 -> Bus Creator/1
  GbWSM_ACWkUpPrs_flg/1 -> Bus Creator/2
  GbWSM_DCWkUpPrs_flg/1 -> Bus Creator/3
  GbWSM_EDCWkUpPrs_flg/1 -> Bus Creator/4
  GeVDP_DriveRqst_enum/1 -> Bus Creator/5
  GeCTC_CtrCtlState_enum/1 -> Bus Creator/6
  GbWSM_TplWkUpPrs_flg/1 -> Bus Creator/7
  GbISP_TFThmRnwyfDet_flg/1 -> Bus Creator/8
  Bus Creator/1 -> Bus Selector1/1, Bus Selector/1
  NoWakeupDelay/1(LbMSM_NoWakeupNetWorkRls_flg) -> Logical Operator3/1
  OnlyTPLWakeup/1(LbMSM_TplWakeupNetWorkRls_flg) -> Logical Operator3/2
  Bus Selector/1 -> NoWakeupDelay/1(GbWSM_Kl15WkUpPrs_flg)  "<GbWSM_Kl15WkUpPrs_flg>"
  Bus Selector/2 -> NoWakeupDelay/2(GbWSM_ACWkUpPrs_flg)  "<GbWSM_ACWkUpPrs_flg>"
  Bus Selector/3 -> NoWakeupDelay/3(GbWSM_DCWkUpPrs_flg)  "<GbWSM_DCWkUpPrs_flg>"
  Bus Selector/4 -> NoWakeupDelay/4(GbWSM_EDCWkUpPrs_flg)  "<GbWSM_EDCWkUpPrs_flg>"
  Bus Selector/5 -> NoWakeupDelay/5(GeVDP_DriveRqst_enum)  "<GeVDP_DriveRqst_enum>"
  Bus Selector/6 -> NoWakeupDelay/6(GeCTC_CtrCtlState_enum)  "<GeCTC_CtrCtlState_enum>"
  Bus Selector/7 -> NoWakeupDelay/7(GbWSM_TplWkUpPrs_flg)  "<GbWSM_TplWkUpPrs_flg>"
  Bus Selector1/1 -> OnlyTPLWakeup/1(GbWSM_Kl15WkUpPrs_flg)  "<GbWSM_Kl15WkUpPrs_flg>"
  Bus Selector1/2 -> OnlyTPLWakeup/2(GbWSM_ACWkUpPrs_flg)  "<GbWSM_ACWkUpPrs_flg>"
  Bus Selector1/3 -> OnlyTPLWakeup/3(GbWSM_DCWkUpPrs_flg)  "<GbWSM_DCWkUpPrs_flg>"
  Bus Selector1/4 -> OnlyTPLWakeup/4(GbWSM_EDCWkUpPrs_flg)  "<GbWSM_EDCWkUpPrs_flg>"
  Bus Selector1/5 -> OnlyTPLWakeup/5(GeVDP_DriveRqst_enum)  "<GeVDP_DriveRqst_enum>"
  Bus Selector1/6 -> OnlyTPLWakeup/6(GeCTC_CtrCtlState_enum)  "<GeCTC_CtrCtlState_enum>"
  Bus Selector1/7 -> OnlyTPLWakeup/7(GbWSM_TplWkUpPrs_flg)  "<GbWSM_TplWkUpPrs_flg>"
  Bus Selector1/8 -> OnlyTPLWakeup/8(GbISP_TFThmRnwyfDet_flg)  "<GbISP_TFThmRnwyfDet_flg>"

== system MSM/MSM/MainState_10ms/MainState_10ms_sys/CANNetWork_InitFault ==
  GeISP_NetWkUpSt_enum : Inport
  Constant9 : Constant  Value=Enum_ISPNetWkUpSt.Enum_ISPNetWkUpSt_UnInit
  Data Type Conversion2 : DataTypeConversion
  MSM_GbMSM_NetWorkUnInitFlt_flg : AIWAYS_Powertrain_BMS_lib/Signals/OverWrite  OverWrite_Value=CbMSM_NetWorkUnInitFltOvr_flg  OverWrite_flag=CbMSM_NetWorkUnInitFltOvrSwt_flg
  Relational Operator5 : RelationalOperator  Operator===  OutDataTypeStr=boolean
  GbMSM_NetWorkUnInitFlt_flg : Outport
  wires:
  Constant9/1 -> Relational Operator5/2
  GeISP_NetWkUpSt_enum/1 -> Data Type Conversion2/1
  Data Type Conversion2/1 -> Relational Operator5/1
  Relational Operator5/1 -> MSM_GbMSM_NetWorkUnInitFlt_flg/1
  MSM_GbMSM_NetWorkUnInitFlt_flg/1 -> GbMSM_NetWorkUnInitFlt_flg/1  "GbMSM_NetWorkUnInitFlt_flg"

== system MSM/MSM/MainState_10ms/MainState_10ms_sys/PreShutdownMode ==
  GaCDP_CellBalc_flg : Inport
  Enable : EnablePort  StatesWhenEnabling=reset
  PreShutdownToShutdownCondition : Subsystem
  LbMSM_PreShutToShut_flg : Outport
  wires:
  PreShutdownToShutdownCondition/1(LbMSM_PreShutToShut_flg) -> LbMSM_PreShutToShut_flg/1
  GaCDP_CellBalc_flg/1 -> PreShutdownToShutdownCondition/1(GaCDP_CellBalc_flg)

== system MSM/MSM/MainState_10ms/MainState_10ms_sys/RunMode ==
  GbWSM_CANWkUpPrs_flg : Inport
  Enable : EnablePort  StatesWhenEnabling=reset
  Constant : Constant  Value=ASWTYPE_FALSE
  Relational Operator2 : RelationalOperator  Operator===  OutDataTypeStr=boolean
  LbMSM_RunToPreShut_flg : Outport
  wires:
  Constant/1 -> Relational Operator2/2
  Relational Operator2/1 -> LbMSM_RunToPreShut_flg/1  "LbMSM_RunToPreShut_flg"
  GbWSM_CANWkUpPrs_flg/1 -> Relational Operator2/1

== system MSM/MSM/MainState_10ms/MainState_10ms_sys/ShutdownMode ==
  GcWSM_WakeupSrc_numb : Inport
  GeISP_NetWkUpSt_enum : Inport  Port=2
  Enable : EnablePort  StatesWhenEnabling=reset
  ShutdownToStandbyCondition : Subsystem
  LbMSM_ShutdownToStb_flg : Outport
  LbMSM_SleepReq_flg : Outport  Port=2
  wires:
  ShutdownToStandbyCondition/1(LbMSM_ShutdownToStb_flg) -> LbMSM_ShutdownToStb_flg/1
  GcWSM_WakeupSrc_numb/1 -> ShutdownToStandbyCondition/1(GcWSM_WakeupSrc_numb)
  ShutdownToStandbyCondition/2(LbMSM_SleepReq_flg) -> LbMSM_SleepReq_flg/1
  GeISP_NetWkUpSt_enum/1 -> ShutdownToStandbyCondition/2(GeISP_NetWkUpSt_enum)

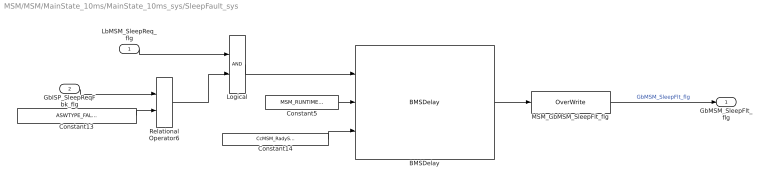
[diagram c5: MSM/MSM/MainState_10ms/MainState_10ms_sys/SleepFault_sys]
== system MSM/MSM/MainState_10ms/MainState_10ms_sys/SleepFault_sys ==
  LbMSM_SleepReq_flg : Inport
  GbISP_SleepReqFbk_flg : Inport  Port=2
  BMSDelay : AIWAYS_Powertrain_BMS_lib/Debounce & Delay/BMSDelay
  Constant13 : Constant  Value=ASWTYPE_FALSE
  Constant14 : Constant  Value=CcMSM_RadySleepFltTi_ms
  Constant5 : Constant  Value=MSM_RUNTIME_MS
  Logical : Logic  OutDataTypeStr=boolean
  MSM_GbMSM_SleepFlt_flg : AIWAYS_Powertrain_BMS_lib/Signals/OverWrite  OverWrite_Value=CbMSM_SleepFltOvr_flg  OverWrite_flag=CbMSM_SleepFltOvrSwt_flg
  Relational Operator6 : RelationalOperator  Operator===  OutDataTypeStr=boolean
  GbMSM_SleepFlt_flg : Outport
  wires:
  LbMSM_SleepReq_flg/1 -> Logical/1
  Constant13/1 -> Relational Operator6/2
  Constant5/1 -> BMSDelay/2
  Constant14/1 -> BMSDelay/3
  Relational Operator6/1 -> Logical/2
  Logical/1 -> BMSDelay/1
  BMSDelay/1 -> MSM_GbMSM_SleepFlt_flg/1
  MSM_GbMSM_SleepFlt_flg/1 -> GbMSM_SleepFlt_flg/1  "GbMSM_SleepFlt_flg"
  GbISP_SleepReqFbk_flg/1 -> Relational Operator6/1

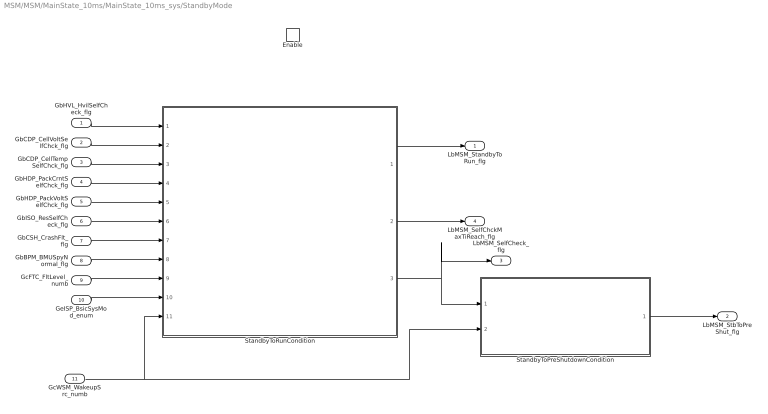
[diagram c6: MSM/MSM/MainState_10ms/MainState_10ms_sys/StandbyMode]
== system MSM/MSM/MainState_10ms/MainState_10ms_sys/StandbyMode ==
  GbHVL_HvilSelfCheck_flg : Inport
  GbCDP_CellVoltSelfChck_flg : Inport  Port=2
  GbCDP_CellTempSelfChck_flg : Inport  Port=3
  GbHDP_PackCrntSelfChck_flg : Inport  Port=4
  GbHDP_PackVoltSelfChck_flg : Inport  Port=5
  GbISO_ResSelfCheck_flg : Inport  Port=6
  GbCSH_CrashFlt_flg : Inport  Port=7
  GbBPM_BMUSpyNormal_flg : Inport  Port=8
  GcFTC_FltLevel_numb : Inport  Port=9
  GeISP_BsicSysMod_enum : Inport  Port=10
  GcWSM_WakeupSrc_numb : Inport  Port=11
  Enable : EnablePort  StatesWhenEnabling=reset
  StandbyToPreShutdownCondition : Subsystem
  StandbyToRunCondition : Subsystem
  LbMSM_StandbyToRun_flg : Outport
  LbMSM_StbToPreShut_flg : Outport  Port=2
  LbMSM_SelfCheck_flg : Outport  Port=3
  LbMSM_SelfChckMaxTiReach_flg : Outport  Port=4
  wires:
  StandbyToRunCondition/1(LbMSM_StandbyToRun_flg) -> LbMSM_StandbyToRun_flg/1
  StandbyToPreShutdownCondition/1(LbMSM_StbToPreShut_flg) -> LbMSM_StbToPreShut_flg/1
  GbHVL_HvilSelfCheck_flg/1 -> StandbyToRunCondition/1(GbHVL_HvilSelfCheck_flg)
  GbCDP_CellVoltSelfChck_flg/1 -> StandbyToRunCondition/2(GbCDP_CellVoltSelfChck_flg)
  GbCDP_CellTempSelfChck_flg/1 -> StandbyToRunCondition/3(GbCDP_CellTempSelfChck_flg)
  GbHDP_PackCrntSelfChck_flg/1 -> StandbyToRunCondition/4(GbHDP_PackCrntSelfChck_flg)
  GbHDP_PackVoltSelfChck_flg/1 -> StandbyToRunCondition/5(GbHDP_PackVoltSelfChck_flg)
  GbISO_ResSelfCheck_flg/1 -> StandbyToRunCondition/6(GbISO_ResSelfCheck_flg)
  GbCSH_CrashFlt_flg/1 -> StandbyToRunCondition/7(GbCSH_CrashFlt_flg)
  GbBPM_BMUSpyNormal_flg/1 -> StandbyToRunCondition/8(GbBPM_BMUSpyNormal_flg)
  GcFTC_FltLevel_numb/1 -> StandbyToRunCondition/9(GcFTC_FltLevel_numb)
  GeISP_BsicSysMod_enum/1 -> StandbyToRunCondition/10(GeISP_BsicSysMod_enum)
  GcWSM_WakeupSrc_numb/1 -> StandbyToPreShutdownCondition/2(GcWSM_WakeupSrc_numb), StandbyToRunCondition/11(GcWSM_WakeupSrc_numb)
  StandbyToRunCondition/3(LbMSM_SelfCheck_flg) -> LbMSM_SelfCheck_flg/1, StandbyToPreShutdownCondition/1(LbMSM_SelfCheck_flg)
  StandbyToRunCondition/2(LbMSM_SelfChckMaxTiReach_flg) -> LbMSM_SelfChckMaxTiReach_flg/1

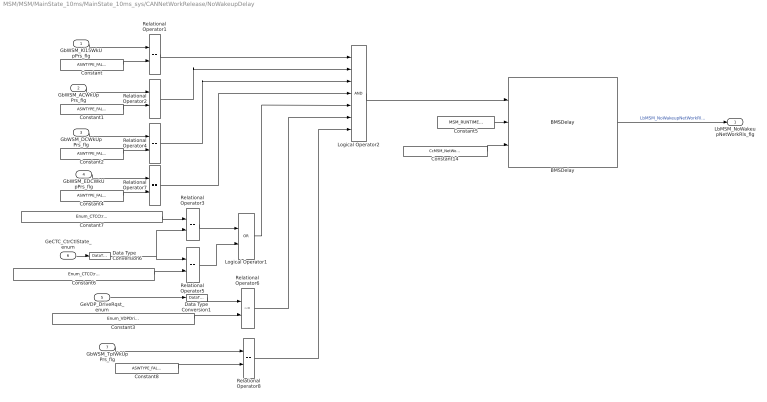
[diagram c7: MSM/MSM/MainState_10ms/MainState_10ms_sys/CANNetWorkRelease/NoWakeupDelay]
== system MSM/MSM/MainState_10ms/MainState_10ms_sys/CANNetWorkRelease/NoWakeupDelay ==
  GbWSM_Kl15WkUpPrs_flg : Inport
  GbWSM_ACWkUpPrs_flg : Inport  Port=2
  GbWSM_DCWkUpPrs_flg : Inport  Port=3
  GbWSM_EDCWkUpPrs_flg : Inport  Port=4
  GeVDP_DriveRqst_enum : Inport  Port=5
  GeCTC_CtrCtlState_enum : Inport  Port=6
  GbWSM_TplWkUpPrs_flg : Inport  Port=7
  BMSDelay : AIWAYS_Powertrain_BMS_lib/Debounce & Delay/BMSDelay
  Constant{,1..2,4,8} (5 alike) : Constant  Value=ASWTYPE_FALSE
  Constant14 : Constant  Value=CcMSM_NetWorkRlsTi_ms
  Constant3 : Constant  Value=Enum_VDPDriveRqst.Enum_VDPDriveRqst_PowerUp
  Constant5 : Constant  Value=MSM_RUNTIME_MS
  Constant6 : Constant  Value=Enum_CTCCtrCtlState.Enum_CTCCtrCtlState_Offline
  Constant7 : Constant  Value=Enum_CTCCtrCtlState.Enum_CTCCtrCtlState_Shutdown
  Data Type Conversion1 : DataTypeConversion
  Data Type Conversion6 : DataTypeConversion
  Logical Operator1 : Logic  Operator=OR  AllPortsSameDT=off  OutDataTypeStr=boolean
  Logical Operator2 : Logic  Inputs=7  AllPortsSameDT=off  OutDataTypeStr=boolean
  Relational Operator{1..5,7..8} (7 alike) : RelationalOperator  Operator===  OutDataTypeStr=boolean
  Relational Operator6 : RelationalOperator  Operator=~=  OutDataTypeStr=boolean
  LbMSM_NoWakeupNetWorkRls_flg : Outport
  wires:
  Constant8/1 -> Relational Operator8/2
  Constant1/1 -> Relational Operator2/2
  Relational Operator2/1 -> Logical Operator2/2
  Constant4/1 -> Relational Operator7/2
  Constant3/1 -> Relational Operator6/2
  Data Type Conversion6/1 -> Relational Operator3/2, Relational Operator5/1
  Relational Operator3/1 -> Logical Operator1/1
  Relational Operator1/1 -> Logical Operator2/1
  Data Type Conversion1/1 -> Relational Operator6/1
  Constant2/1 -> Relational Operator4/2
  Constant6/1 -> Relational Operator5/2
  Constant7/1 -> Relational Operator3/1
  Constant/1 -> Relational Operator1/2
  Relational Operator6/1 -> Logical Operator2/6
  Relational Operator5/1 -> Logical Operator1/2
  Logical Operator1/1 -> Logical Operator2/5
  Relational Operator4/1 -> Logical Operator2/3
  Relational Operator7/1 -> Logical Operator2/4
  GeCTC_CtrCtlState_enum/1 -> Data Type Conversion6/1
  GbWSM_DCWkUpPrs_flg/1 -> Relational Operator4/1
  Relational Operator8/1 -> Logical Operator2/7
  GbWSM_EDCWkUpPrs_flg/1 -> Relational Operator7/1
  GeVDP_DriveRqst_enum/1 -> Data Type Conversion1/1
  GbWSM_TplWkUpPrs_flg/1 -> Relational Operator8/1
  GbWSM_Kl15WkUpPrs_flg/1 -> Relational Operator1/1
  GbWSM_ACWkUpPrs_flg/1 -> Relational Operator2/1
  Constant5/1 -> BMSDelay/2
  Constant14/1 -> BMSDelay/3
  Logical Operator2/1 -> BMSDelay/1
  BMSDelay/1 -> LbMSM_NoWakeupNetWorkRls_flg/1  "LbMSM_NoWakeupNetWorkRls_flg"

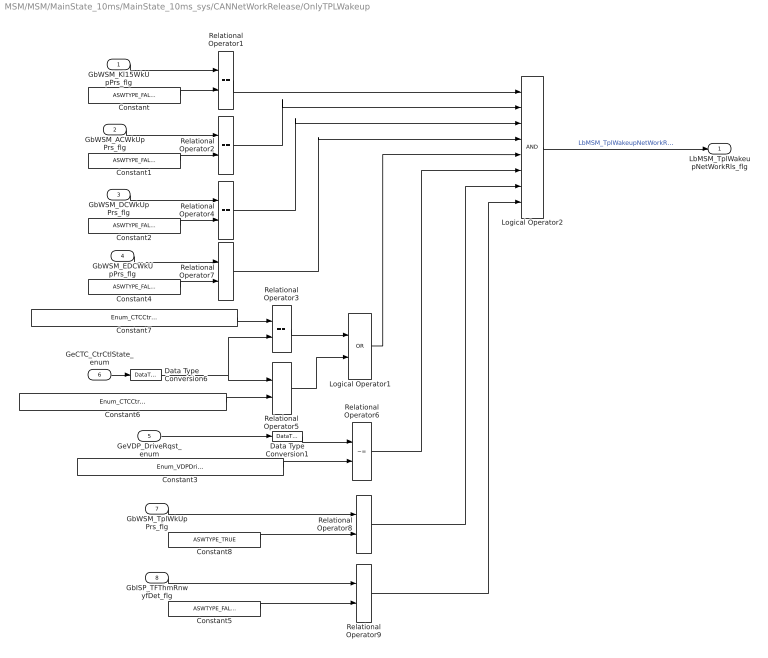
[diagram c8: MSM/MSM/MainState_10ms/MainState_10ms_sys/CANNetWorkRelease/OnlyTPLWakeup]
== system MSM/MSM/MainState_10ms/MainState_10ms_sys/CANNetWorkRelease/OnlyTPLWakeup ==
  GbWSM_Kl15WkUpPrs_flg : Inport
  GbWSM_ACWkUpPrs_flg : Inport  Port=2
  GbWSM_DCWkUpPrs_flg : Inport  Port=3
  GbWSM_EDCWkUpPrs_flg : Inport  Port=4
  GeVDP_DriveRqst_enum : Inport  Port=5
  GeCTC_CtrCtlState_enum : Inport  Port=6
  GbWSM_TplWkUpPrs_flg : Inport  Port=7
  GbISP_TFThmRnwyfDet_flg : Inport  Port=8
  Constant{,1..2,4..5} (5 alike) : Constant  Value=ASWTYPE_FALSE
  Constant3 : Constant  Value=Enum_VDPDriveRqst.Enum_VDPDriveRqst_PowerUp
  Constant6 : Constant  Value=Enum_CTCCtrCtlState.Enum_CTCCtrCtlState_Offline
  Constant7 : Constant  Value=Enum_CTCCtrCtlState.Enum_CTCCtrCtlState_Shutdown
  Constant8 : Constant  Value=ASWTYPE_TRUE
  Data Type Conversion1 : DataTypeConversion
  Data Type Conversion6 : DataTypeConversion
  Logical Operator1 : Logic  Operator=OR  AllPortsSameDT=off  OutDataTypeStr=boolean
  Logical Operator2 : Logic  Inputs=8  AllPortsSameDT=off  OutDataTypeStr=boolean
  Relational Operator{1..5,7..9} (8 alike) : RelationalOperator  Operator===  OutDataTypeStr=boolean
  Relational Operator6 : RelationalOperator  Operator=~=  OutDataTypeStr=boolean
  LbMSM_TplWakeupNetWorkRls_flg : Outport
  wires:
  GbWSM_ACWkUpPrs_flg/1 -> Relational Operator2/1
  GbWSM_Kl15WkUpPrs_flg/1 -> Relational Operator1/1
  GbWSM_TplWkUpPrs_flg/1 -> Relational Operator8/1
  GeVDP_DriveRqst_enum/1 -> Data Type Conversion1/1
  GbWSM_EDCWkUpPrs_flg/1 -> Relational Operator7/1
  Relational Operator8/1 -> Logical Operator2/7
  GbWSM_DCWkUpPrs_flg/1 -> Relational Operator4/1
  GeCTC_CtrCtlState_enum/1 -> Data Type Conversion6/1
  Relational Operator7/1 -> Logical Operator2/4
  Relational Operator4/1 -> Logical Operator2/3
  Logical Operator1/1 -> Logical Operator2/5
  Relational Operator5/1 -> Logical Operator1/2
  Relational Operator6/1 -> Logical Operator2/6
  Constant/1 -> Relational Operator1/2
  Constant7/1 -> Relational Operator3/1
  Constant6/1 -> Relational Operator5/2
  Constant2/1 -> Relational Operator4/2
  Data Type Conversion1/1 -> Relational Operator6/1
  Relational Operator1/1 -> Logical Operator2/1
  Relational Operator3/1 -> Logical Operator1/1
  Data Type Conversion6/1 -> Relational Operator5/1, Relational Operator3/2
  Constant3/1 -> Relational Operator6/2
  Constant4/1 -> Relational Operator7/2
  Relational Operator2/1 -> Logical Operator2/2
  Constant1/1 -> Relational Operator2/2
  Constant8/1 -> Relational Operator8/2
  Constant5/1 -> Relational Operator9/2
  GbISP_TFThmRnwyfDet_flg/1 -> Relational Operator9/1
  Relational Operator9/1 -> Logical Operator2/8
  Logical Operator2/1 -> LbMSM_TplWakeupNetWorkRls_flg/1  "LbMSM_TplWakeupNetWorkRls_flg"

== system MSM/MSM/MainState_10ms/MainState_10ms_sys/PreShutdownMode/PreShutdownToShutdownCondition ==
  GaCDP_CellBalc_flg : Inport
  BMSDelay : AIWAYS_Powertrain_BMS_lib/Debounce & Delay/BMSDelay
  Constant : Constant  Value=ASWTYPE_FALSE
  Constant1 : Constant  Value=CcMSM_PreShutTi_ms
  Constant3 : Constant  Value=MSM_RUNTIME_MS
  Constant4 : Constant  Value=ASWTYPE_TRUE
  Logical Operator1 : Logic  Operator=OR  Inputs=1  AllPortsSameDT=off  OutDataTypeStr=boolean
  Logical Operator3 : Logic  Operator=OR  AllPortsSameDT=off  OutDataTypeStr=boolean
  Relational Operator6 : RelationalOperator  Operator===  OutDataTypeStr=boolean
  LbMSM_PreShutToShut_flg : Outport
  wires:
  Logical Operator3/1 -> LbMSM_PreShutToShut_flg/1  "LbMSM_PreShutToShut_flg"
  GaCDP_CellBalc_flg/1 -> Logical Operator1/1
  Constant/1 -> Relational Operator6/2
  BMSDelay/1 -> Logical Operator3/1
  Relational Operator6/1 -> Logical Operator3/2
  Logical Operator1/1 -> Relational Operator6/1
  Constant3/1 -> BMSDelay/2
  Constant1/1 -> BMSDelay/3
  Constant4/1 -> BMSDelay/1

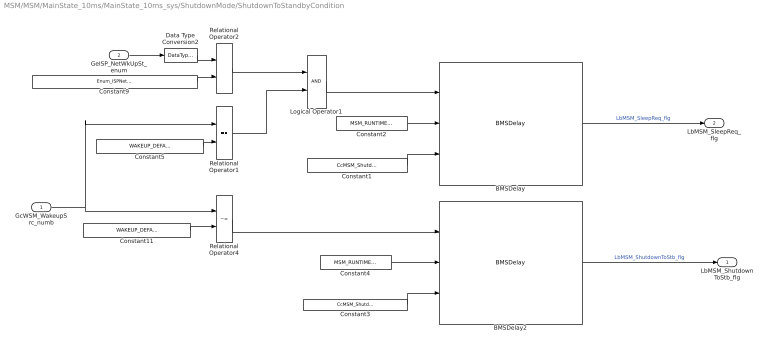
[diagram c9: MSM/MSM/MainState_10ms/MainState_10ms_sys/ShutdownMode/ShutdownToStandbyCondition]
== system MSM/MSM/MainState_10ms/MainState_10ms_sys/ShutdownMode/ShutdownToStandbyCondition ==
  GcWSM_WakeupSrc_numb : Inport
  GeISP_NetWkUpSt_enum : Inport  Port=2
  BMSDelay : AIWAYS_Powertrain_BMS_lib/Debounce & Delay/BMSDelay
  BMSDelay2 : AIWAYS_Powertrain_BMS_lib/Debounce & Delay/BMSDelay
  Constant1 : Constant  Value=CcMSM_ShutdownToSleepTi_ms
  Constant11 : Constant  Value=WAKEUP_DEFAULT
  Constant2 : Constant  Value=MSM_RUNTIME_MS
  Constant3 : Constant  Value=CcMSM_ShutdownToStbTi_ms
  Constant4 : Constant  Value=MSM_RUNTIME_MS
  Constant5 : Constant  Value=WAKEUP_DEFAULT
  Constant9 : Constant  Value=Enum_ISPNetWkUpSt.Enum_ISPNetWkUpSt_BusSleep
  Data Type Conversion2 : DataTypeConversion
  Logical Operator1 : Logic  AllPortsSameDT=off  OutDataTypeStr=boolean
  Relational Operator1 : RelationalOperator  Operator===  OutDataTypeStr=boolean
  Relational Operator2 : RelationalOperator  Operator===  OutDataTypeStr=boolean
  Relational Operator4 : RelationalOperator  Operator=~=  OutDataTypeStr=boolean
  LbMSM_ShutdownToStb_flg : Outport
  LbMSM_SleepReq_flg : Outport  Port=2
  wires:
  BMSDelay2/1 -> LbMSM_ShutdownToStb_flg/1  "LbMSM_ShutdownToStb_flg"
  Constant4/1 -> BMSDelay2/2
  Constant3/1 -> BMSDelay2/3
  Constant2/1 -> BMSDelay/2
  Constant1/1 -> BMSDelay/3
  Relational Operator4/1 -> BMSDelay2/1
  GcWSM_WakeupSrc_numb/1 -> Relational Operator1/1, Relational Operator4/1
  Constant11/1 -> Relational Operator4/2
  Constant5/1 -> Relational Operator1/2
  Constant9/1 -> Relational Operator2/2
  GeISP_NetWkUpSt_enum/1 -> Data Type Conversion2/1
  Data Type Conversion2/1 -> Relational Operator2/1
  Logical Operator1/1 -> BMSDelay/1
  Relational Operator2/1 -> Logical Operator1/1
  Relational Operator1/1 -> Logical Operator1/2
  BMSDelay/1 -> LbMSM_SleepReq_flg/1  "LbMSM_SleepReq_flg"

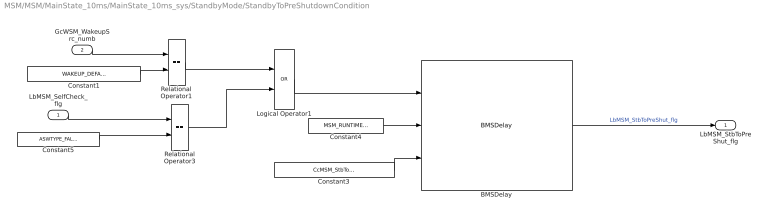
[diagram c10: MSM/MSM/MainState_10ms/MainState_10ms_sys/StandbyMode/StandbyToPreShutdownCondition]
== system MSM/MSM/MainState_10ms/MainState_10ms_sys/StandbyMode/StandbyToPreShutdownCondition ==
  LbMSM_SelfCheck_flg : Inport
  GcWSM_WakeupSrc_numb : Inport  Port=2
  BMSDelay : AIWAYS_Powertrain_BMS_lib/Debounce & Delay/BMSDelay
  Constant1 : Constant  Value=WAKEUP_DEFAULT
  Constant3 : Constant  Value=CcMSM_StbToPreShutDlyTi_ms
  Constant4 : Constant  Value=MSM_RUNTIME_MS
  Constant5 : Constant  Value=ASWTYPE_FALSE
  Logical Operator1 : Logic  Operator=OR  AllPortsSameDT=off  OutDataTypeStr=boolean
  Relational Operator1 : RelationalOperator  Operator===  OutDataTypeStr=boolean
  Relational Operator3 : RelationalOperator  Operator===  OutDataTypeStr=boolean
  LbMSM_StbToPreShut_flg : Outport
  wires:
  BMSDelay/1 -> LbMSM_StbToPreShut_flg/1  "LbMSM_StbToPreShut_flg"
  GcWSM_WakeupSrc_numb/1 -> Relational Operator1/1
  Constant1/1 -> Relational Operator1/2
  Constant4/1 -> BMSDelay/2
  Constant3/1 -> BMSDelay/3
  Constant5/1 -> Relational Operator3/2
  LbMSM_SelfCheck_flg/1 -> Relational Operator3/1
  Relational Operator1/1 -> Logical Operator1/1
  Relational Operator3/1 -> Logical Operator1/2
  Logical Operator1/1 -> BMSDelay/1

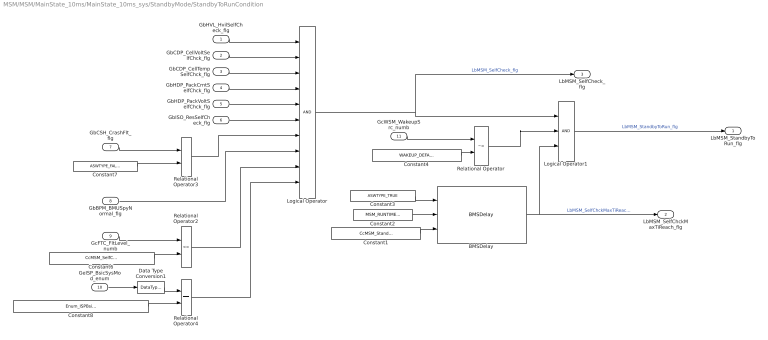
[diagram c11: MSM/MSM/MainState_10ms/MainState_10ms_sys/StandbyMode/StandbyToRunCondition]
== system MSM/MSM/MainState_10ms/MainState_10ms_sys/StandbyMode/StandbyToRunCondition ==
  GbHVL_HvilSelfCheck_flg : Inport
  GbCDP_CellVoltSelfChck_flg : Inport  Port=2
  GbCDP_CellTempSelfChck_flg : Inport  Port=3
  GbHDP_PackCrntSelfChck_flg : Inport  Port=4
  GbHDP_PackVoltSelfChck_flg : Inport  Port=5
  GbISO_ResSelfCheck_flg : Inport  Port=6
  GbCSH_CrashFlt_flg : Inport  Port=7
  GbBPM_BMUSpyNormal_flg : Inport  Port=8
  GcFTC_FltLevel_numb : Inport  Port=9
  GeISP_BsicSysMod_enum : Inport  Port=10
  GcWSM_WakeupSrc_numb : Inport  Port=11
  BMSDelay : AIWAYS_Powertrain_BMS_lib/Debounce & Delay/BMSDelay
  Constant1 : Constant  Value=CcMSM_StandbyRunTime_ms
  Constant2 : Constant  Value=MSM_RUNTIME_MS
  Constant3 : Constant  Value=ASWTYPE_TRUE
  Constant4 : Constant  Value=WAKEUP_DEFAULT
  Constant6 : Constant  Value=CcMSM_SelfCheckFltThrhd_numb
  Constant7 : Constant  Value=ASWTYPE_FALSE
  Constant8 : Constant  Value=Enum_ISPBsicSysMod.Enum_ISPBsicSysMod_Run
  Data Type Conversion1 : DataTypeConversion
  Logical Operator : Logic  Inputs=10  AllPortsSameDT=off  OutDataTypeStr=boolean
  Logical Operator1 : Logic  Inputs=3  AllPortsSameDT=off  OutDataTypeStr=boolean
  Relational Operator : RelationalOperator  Operator=~=  OutDataTypeStr=boolean
  Relational Operator2 : RelationalOperator  Operator=<=  OutDataTypeStr=boolean
  Relational Operator3 : RelationalOperator  Operator===  OutDataTypeStr=boolean
  Relational Operator4 : RelationalOperator  Operator===  OutDataTypeStr=boolean
  LbMSM_StandbyToRun_flg : Outport
  LbMSM_SelfChckMaxTiReach_flg : Outport  Port=2
  LbMSM_SelfCheck_flg : Outport  Port=3
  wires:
  Logical Operator1/1 -> LbMSM_StandbyToRun_flg/1  "LbMSM_StandbyToRun_flg"
  Constant2/1 -> BMSDelay/2
  Constant1/1 -> BMSDelay/3
  Constant3/1 -> BMSDelay/1
  Constant4/1 -> Relational Operator/2
  Data Type Conversion1/1 -> Relational Operator4/1
  GeISP_BsicSysMod_enum/1 -> Data Type Conversion1/1
  Constant8/1 -> Relational Operator4/2
  GbCDP_CellVoltSelfChck_flg/1 -> Logical Operator/2
  Relational Operator4/1 -> Logical Operator/10
  Constant6/1 -> Relational Operator2/2
  GbHDP_PackCrntSelfChck_flg/1 -> Logical Operator/4
  GbISO_ResSelfCheck_flg/1 -> Logical Operator/6
  GcFTC_FltLevel_numb/1 -> Relational Operator2/1
  GbCDP_CellTempSelfChck_flg/1 -> Logical Operator/3
  GbCSH_CrashFlt_flg/1 -> Relational Operator3/1
  GbHDP_PackVoltSelfChck_flg/1 -> Logical Operator/5
  Relational Operator2/1 -> Logical Operator/9
  GbHVL_HvilSelfCheck_flg/1 -> Logical Operator/1
  GbBPM_BMUSpyNormal_flg/1 -> Logical Operator/8
  Relational Operator3/1 -> Logical Operator/7
  Constant7/1 -> Relational Operator3/2
  Logical Operator/1 -> Logical Operator1/1, LbMSM_SelfCheck_flg/1  "LbMSM_SelfCheck_flg"
  GcWSM_WakeupSrc_numb/1 -> Relational Operator/1
  Relational Operator/1 -> Logical Operator1/2
  BMSDelay/1 -> LbMSM_SelfChckMaxTiReach_flg/1, Logical Operator1/3  "LbMSM_SelfChckMaxTiReach_flg"

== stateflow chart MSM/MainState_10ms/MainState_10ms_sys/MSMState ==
  state Standby
    en:
    GeMSM_BMUState_enum = Enum_MSMBMUState.Enum_MSMBMUState_Standby;
  state Run
    en:
    GeMSM_BMUState_enum = Enum_MSMBMUState.Enum_MSMBMUState_Run;
  state Pershutdown
    en:
    GeMSM_BMUState_enum = Enum_MSMBMUState.Enum_MSMBMUState_PreShutdown;
  state Shutdown
    en:
    GeMSM_BMUState_enum = Enum_MSMBMUState.Enum_MSMBMUState_Shutdown;
  (default) -> Standby
  Standby -> Pershutdown : [ASWTYPE_TRUE == LbMSM_StbToPreShut_flg]
  Shutdown -> Standby : [ASWTYPE_TRUE == LbMSM_ShutdownToStb_flg]
  Standby -> Run : [ASWTYPE_TRUE == LbMSM_StandbyToRun_flg]
  Run -> Pershutdown : [ASWTYPE_TRUE == LbMSM_RunToPreShut_flg]
  Pershutdown -> Shutdown : [ASWTYPE_TRUE == LbMSM_PreShutToShut_flg]
  data: LbMSM_StandbyToRun_flg input; LbMSM_StbToPreShut_flg input; GeMSM_BMUState_enum output; LbMSM_RunToPreShut_flg input; LbMSM_PreShutToShut_flg input; LbMSM_ShutdownToStb_flg input; ASWTYPE_TRUE parameter
